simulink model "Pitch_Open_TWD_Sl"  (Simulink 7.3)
settings: Solver=ode45  StartTime=0.0  StopTime=20  RelTol=1e-3
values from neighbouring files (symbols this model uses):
  Aac = [    [actuator_srb.m]    (also in actuator_ssme.m; actuators_5s.m; actuators_5z.m)
  Bac = [    [actuator_srb.m]    (also in actuator_ssme.m; actuators_5s.m; actuators_5z.m)
  Cac = [    [actuator_srb.m]    (also in actuator_ssme.m; actuators_5s.m; actuators_5z.m)
  Dac = [    [actuator_srb.m]    (also in actuator_ssme.m; actuators_5s.m; actuators_5z.m)
undefined symbols (not defined in the file or in its folder): Asb, Ats, Bsb, Bts, Csb, Cts, Dsb, Dts

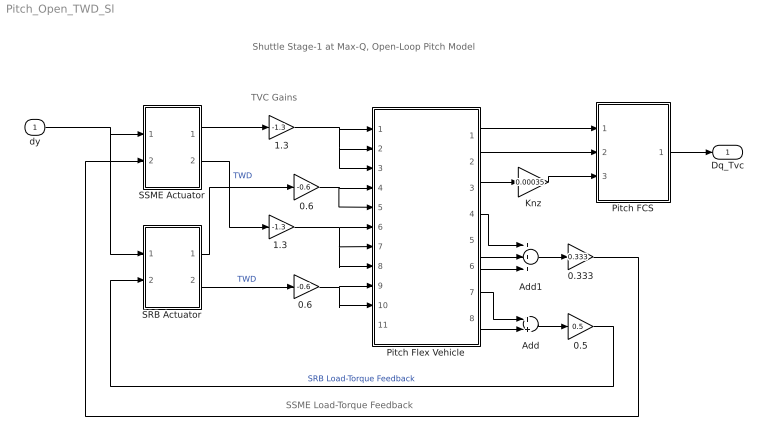
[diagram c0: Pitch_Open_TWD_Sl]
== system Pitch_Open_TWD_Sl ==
  note: SSME Load-Torque Feedback
  note: TVC Gains
  note: Shuttle Stage-1 at Max-Q, Open-Loop Pitch Model
  dy : Inport  OutDataType=sfix(16)  OutScaling=2^0
  0.333 : Gain  Gain=0.333  ParameterDataType=sfix(16)  ParameterScaling=2^0  OutDataType=sfix(16)  OutScaling=2^0
  0.5 : Gain  Gain=0.5  ParameterDataType=sfix(16)  ParameterScaling=2^0  OutDataType=sfix(16)  OutScaling=2^0
  0.6 : Gain  Gain=-0.6  ParameterDataType=sfix(16)  ParameterScaling=2^0  OutDataType=sfix(16)  OutScaling=2^0
  "0.6 " : Gain  Gain=-0.6  ParameterDataType=sfix(16)  ParameterScaling=2^0  OutDataType=sfix(16)  OutScaling=2^0
  1.3 : Gain  Gain=-1.3  ParameterDataType=sfix(16)  ParameterScaling=2^0  OutDataType=sfix(16)  OutScaling=2^0
  "1.3 " : Gain  Gain=-1.3  ParameterDataType=sfix(16)  ParameterScaling=2^0  OutDataType=sfix(16)  OutScaling=2^0
  Add : Sum  OutDataType=sfix(16)  OutScaling=2^-10
  Add1 : Sum  Inputs=+++  OutDataType=sfix(16)  OutScaling=2^-10
  Knz : Gain  Gain=0.00035  ParameterDataType=sfix(16)  ParameterScaling=2^0  OutDataType=sfix(16)  OutScaling=2^0
  Pitch FCS : Subsystem
  Pitch Flex Vehicle : Subsystem
  SRB Actuator : Subsystem
  SSME Actuator : Subsystem
  Dq_Tvc : Outport  OutDataType=sfix(16)  OutScaling=2^0
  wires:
  SSME Actuator/1(dy) -> 1.3/1
  dy/1 -> SSME Actuator/1(dy-com), SRB Actuator/1(dy-com)
  1.3/1 -> Pitch Flex Vehicle/1(dy1), Pitch Flex Vehicle/2(dy2), Pitch Flex Vehicle/3(dy3)
  0.6/1 -> Pitch Flex Vehicle/4(dy4), Pitch Flex Vehicle/5(dy5)
  SSME Actuator/2(dy-dd) -> "1.3 "/1  "TWD"
  "1.3 "/1 -> Pitch Flex Vehicle/6(dydd1), Pitch Flex Vehicle/7(dydd2), Pitch Flex Vehicle/8(dydd3)
  "0.6 "/1 -> Pitch Flex Vehicle/9(dydd4), Pitch Flex Vehicle/10(dydd5)
  Pitch Flex Vehicle/1(theta) -> Pitch FCS/1(theta)
  Pitch Flex Vehicle/2(q-rb) -> Pitch FCS/2(q)
  Pitch Flex Vehicle/3(Nz) -> Knz/1
  Knz/1 -> Pitch FCS/3(Nz)
  SRB Actuator/1(dy) -> 0.6/1
  SRB Actuator/2(dy-dd) -> "0.6 "/1  "TWD"
  Pitch Flex Vehicle/7(TLy4) -> Add/1
  Pitch Flex Vehicle/8(TLy5) -> Add/2
  Add/1 -> 0.5/1
  0.5/1 -> SRB Actuator/2(TL)  "SRB Load-Torque Feedback"
  Add1/1 -> 0.333/1
  Pitch Flex Vehicle/6(TLy3) -> Add1/3
  Pitch Flex Vehicle/5(TLy2) -> Add1/2
  Pitch Flex Vehicle/4(TLy1) -> Add1/1
  0.333/1 -> SSME Actuator/2(TL)
  Pitch FCS/1(DQ_TVC) -> Dq_Tvc/1

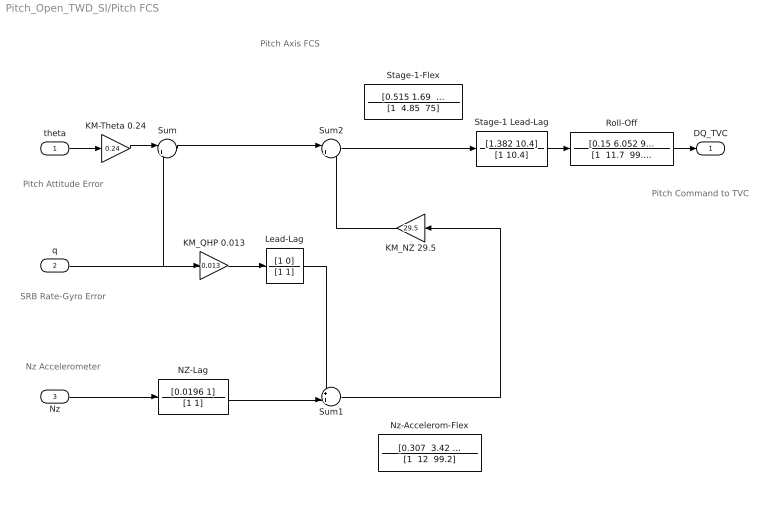
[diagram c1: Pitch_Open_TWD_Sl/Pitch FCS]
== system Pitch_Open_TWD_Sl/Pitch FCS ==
  note: Pitch Command to TVC
  note: SRB Rate-Gyro Error
  note: Pitch Attitude Error
  note: Nz Accelerometer
  note: Pitch Axis FCS
  theta : Inport  OutDataType=fixdt(1, 16)  OutScaling=2^0
  q : Inport  Port=2  OutDataType=fixdt(1, 16)  OutScaling=2^0
  Nz : Inport  Port=3  OutDataType=fixdt(1, 16)  OutScaling=2^0
  KM-Theta 0.24 : Gain  Gain=0.24  ParameterDataType=fixdt(1, 16)  ParameterScaling=2^0  OutDataType=fixdt(1, 16)  OutScaling=2^0
  KM_NZ 29.5 : Gain  Gain=29.5  ParameterDataType=fixdt(1, 16)  ParameterScaling=2^0  OutDataType=fixdt(1, 16)  OutScaling=2^0
  KM_QHP 0.013 : Gain  Gain=0.013  ParameterDataType=fixdt(1, 16)  ParameterScaling=2^0  OutDataType=fixdt(1, 16)  OutScaling=2^0
  Lead-Lag : TransferFcn  Numerator=[1 0]  Denominator=[1 1]
  NZ-Lag : TransferFcn  Numerator=[0.0196 1]  Denominator=[1 1]
  Nz-Accelerom-Flex : TransferFcn  Numerator="[0.307  3.42  99.2]"  Denominator="[1  12  99.2]"
  Roll-Off : TransferFcn  Numerator=[0.15 6.052 99.2]  Denominator="[1  11.7  99.2]"
  Stage-1 Lead-Lag : TransferFcn  Numerator=[1.382 10.4]  Denominator=[1 10.4]
  Stage-1-Flex : TransferFcn  Numerator="[0.515 1.69  75]"  Denominator="[1  4.85  75]"
  Sum : Sum  Inputs=|++  OutDataType=fixdt(1, 16)  OutScaling=2^0
  Sum1 : Sum  Inputs=++|  OutDataType=fixdt(1, 16)  OutScaling=2^0
  Sum2 : Sum  Inputs=|++  OutDataType=fixdt(1, 16)  OutScaling=2^0
  DQ_TVC : Outport  OutDataType=fixdt(1, 16)  OutScaling=2^0
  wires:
  Roll-Off/1 -> DQ_TVC/1
  KM_NZ 29.5/1 -> Sum2/2
  Sum2/1 -> Stage-1 Lead-Lag/1
  Lead-Lag/1 -> Sum1/1
  Sum1/1 -> KM_NZ 29.5/1
  NZ-Lag/1 -> Sum1/2
  Stage-1 Lead-Lag/1 -> Roll-Off/1
  Nz/1 -> NZ-Lag/1
  KM_QHP 0.013/1 -> Lead-Lag/1
  q/1 -> KM_QHP 0.013/1, Sum/2
  Sum/1 -> Sum2/1
  KM-Theta 0.24/1 -> Sum/1
  theta/1 -> KM-Theta 0.24/1

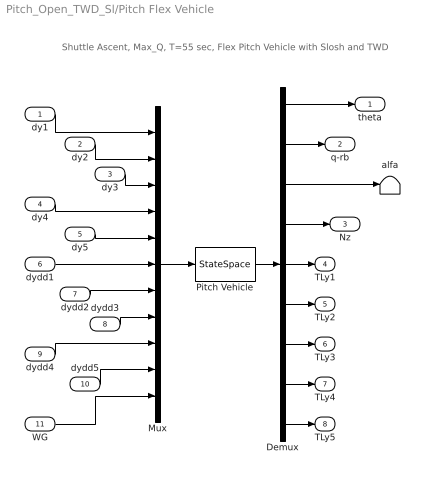
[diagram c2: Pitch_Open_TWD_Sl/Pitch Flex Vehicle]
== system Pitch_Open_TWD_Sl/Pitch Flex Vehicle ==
  note: Shuttle Ascent, Max_Q, T=55 sec, Flex Pitch Vehicle with Slosh and TWD
  dy1 : Inport  OutDataType=sfix(16)  OutScaling=2^0
  dy2 : Inport  Port=2  OutDataType=sfix(16)  OutScaling=2^0
  dy3 : Inport  Port=3  OutDataType=sfix(16)  OutScaling=2^0
  dy4 : Inport  Port=4  OutDataType=sfix(16)  OutScaling=2^0
  dy5 : Inport  Port=5  OutDataType=sfix(16)  OutScaling=2^0
  dydd1 : Inport  Port=6  OutDataType=sfix(16)  OutScaling=2^0
  dydd2 : Inport  Port=7  OutDataType=sfix(16)  OutScaling=2^0
  dydd3 : Inport  Port=8  OutDataType=sfix(16)  OutScaling=2^0
  dydd4 : Inport  Port=9  OutDataType=sfix(16)  OutScaling=2^0
  dydd5 : Inport  Port=10  OutDataType=sfix(16)  OutScaling=2^0
  WG : Inport  Port=11  OutDataType=sfix(16)  OutScaling=2^0
  Demux : Demux  Outputs=9
  Mux : Mux  Inputs=11
  Pitch Vehicle : StateSpace  A=Ats  B=Bts  C=Cts  D=Dts
  alfa : Terminator
  theta : Outport  OutDataType=sfix(16)  OutScaling=2^0
  q-rb : Outport  Port=2  OutDataType=sfix(16)  OutScaling=2^0
  Nz : Outport  Port=3  OutDataType=sfix(16)  OutScaling=2^0
  TLy1 : Outport  Port=4  OutDataType=sfix(16)  OutScaling=2^0
  TLy2 : Outport  Port=5  OutDataType=sfix(16)  OutScaling=2^0
  TLy3 : Outport  Port=6  OutDataType=sfix(16)  OutScaling=2^0
  TLy4 : Outport  Port=7  OutDataType=sfix(16)  OutScaling=2^0
  TLy5 : Outport  Port=8  OutDataType=sfix(16)  OutScaling=2^0
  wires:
  Pitch Vehicle/1 -> Demux/1
  Mux/1 -> Pitch Vehicle/1
  dy1/1 -> Mux/1
  dy2/1 -> Mux/2
  dy3/1 -> Mux/3
  dy4/1 -> Mux/4
  dy5/1 -> Mux/5
  dydd1/1 -> Mux/6
  dydd2/1 -> Mux/7
  dydd3/1 -> Mux/8
  dydd4/1 -> Mux/9
  dydd5/1 -> Mux/10
  WG/1 -> Mux/11
  Demux/1 -> theta/1
  Demux/2 -> q-rb/1
  Demux/3 -> alfa/1
  Demux/4 -> Nz/1
  Demux/5 -> TLy1/1
  Demux/9 -> TLy5/1
  Demux/8 -> TLy4/1
  Demux/7 -> TLy3/1
  Demux/6 -> TLy2/1

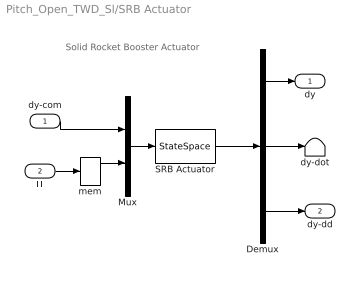
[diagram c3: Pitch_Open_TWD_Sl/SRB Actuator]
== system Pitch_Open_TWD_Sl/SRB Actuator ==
  note: Solid Rocket Booster Actuator
  dy-com : Inport  PortDimensions=1  OutDataType=sfix(16)  OutScaling=2^0
  TL : Inport  Port=2  OutDataType=sfix(16)  OutScaling=2^0
  Demux : Demux  Outputs=3
  Mux : Mux  Inputs=2
  SRB Actuator : StateSpace  A=Asb  B=Bsb  C=Csb  D=Dsb
  dy-dot : Terminator
  mem : Memory
  dy : Outport  OutDataType=sfix(16)  OutScaling=2^0
  dy-dd : Outport  Port=2  OutDataType=sfix(16)  OutScaling=2^0
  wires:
  SRB Actuator/1 -> Demux/1
  Mux/1 -> SRB Actuator/1
  Demux/1 -> dy/1
  dy-com/1 -> Mux/1
  TL/1 -> mem/1
  Demux/2 -> dy-dot/1
  Demux/3 -> dy-dd/1
  mem/1 -> Mux/2

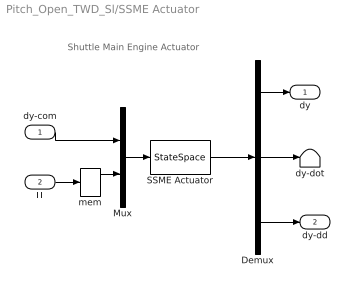
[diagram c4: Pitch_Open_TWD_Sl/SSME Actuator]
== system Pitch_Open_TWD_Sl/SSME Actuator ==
  note: Shuttle Main Engine Actuator
  dy-com : Inport  PortDimensions=1  OutDataType=sfix(16)  OutScaling=2^0
  TL : Inport  Port=2  OutDataType=sfix(16)  OutScaling=2^0
  Demux : Demux  Outputs=3
  Mux : Mux  Inputs=2
  SSME Actuator : StateSpace  A=Aac  B=Bac  C=Cac  D=Dac
  dy-dot : Terminator
  mem : Memory
  dy : Outport  OutDataType=sfix(16)  OutScaling=2^0
  dy-dd : Outport  Port=2  OutDataType=sfix(16)  OutScaling=2^0
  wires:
  SSME Actuator/1 -> Demux/1
  Mux/1 -> SSME Actuator/1
  Demux/1 -> dy/1
  dy-com/1 -> Mux/1
  TL/1 -> mem/1
  Demux/2 -> dy-dot/1
  Demux/3 -> dy-dd/1
  mem/1 -> Mux/2
